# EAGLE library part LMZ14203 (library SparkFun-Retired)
3A, Simple Switcher Power Module with 42V Maximum Input
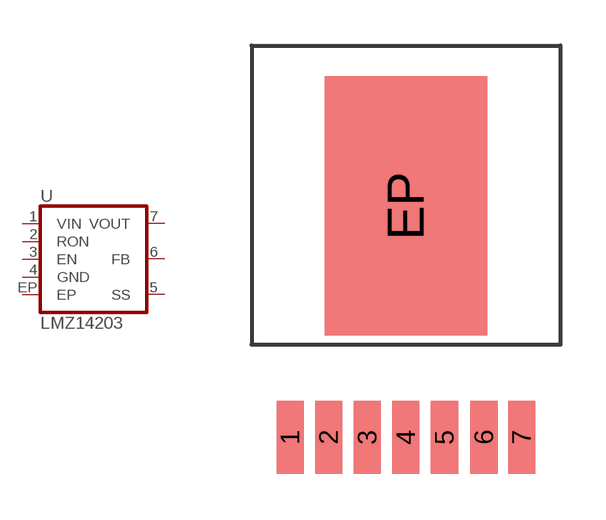
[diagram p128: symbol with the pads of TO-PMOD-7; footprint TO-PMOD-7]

Designator prefix U

## LMZ14203  [TO-PMOD-7]
1  VIN
2  RON
3  EN
4  GND
5  SS
6  FB
7  VOUT
EP  EP

## Footprint TO-PMOD-7 (pad centres in mm)
7-Lead package for National voltage switchers (LMZ14203)
smd 0.89 x 2.41: 1 -3.81,-7.63; 2 -2.54,-7.63; 3 -1.27,-7.63; 4 0,-7.63; 5 1.27,-7.63; 6 2.57,-7.63; 7 3.81,-7.63
smd 5.35 x 8.54: EP 0,0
